(* Logix 5000 AddOnInstructionDefinition export AMCI_5034_PTO_AM_MAFR; software revision 37.00 *)

TYPE AMCI_5034_PTO_AM_Input_Data :
STRUCT
   ConnectionFaulted : DINT;
   MovingCW : BOOL;
   MovingCCW : BOOL;
   InHoldState : BOOL;
   Stopped : BOOL;
   AtHome : BOOL;
   Accelerating : BOOL;
   Decelerating : BOOL;
   MoveComplete : BOOL;
   HomeInvalid : BOOL;
   InvalidProfile : BOOL;
   PositionInvalid : BOOL;
   InputError : BOOL;
   CommandError : BOOL;
   ConfigurationError : BOOL;
   ModuleOK : BOOL;
   GeneralPurposeOutputStatus : BOOL;
   Input1Active : BOOL;
   Input2Active : BOOL;
   Input3Active : BOOL;
   Input4Active : BOOL;
   bit_20_reserved : BOOL;
   bit_21_reserved : BOOL;
   bit_22_reserved : BOOL;
   EncoderFollowerMode : BOOL;
   BlendMoveRunning : BOOL;
   BlendMoveAcknowledge : BOOL;
   MinimumRegistrationProgrammed : BOOL;
   EncoderMotionDirection : BOOL;
   MultipleInputsWithSameFunction : BOOL;
   FSCExceedsNumberOfDataBits : BOOL;
   AbsoluteEncoderSetupError : BOOL;
   bit_31_reserved : BOOL;
   CurrentPosition : DINT;
   EncoderPosition : DINT;
   CapturedPosition : DINT;
END_STRUCT
END_TYPE

TYPE AMCI_5034_PTO_AM_Output_Data :
STRUCT
   Command_Word : DINT;
   TargetPosition : DINT;
   TargetVelocity : UDINT;
   Acceleration : DINT;
   Deceleration : DINT;
END_STRUCT
END_TYPE

ADD_ON_INSTRUCTION AMCI_5034_PTO_AM_MAFR   (* revision 1.0, vendor AMCI, ExecuteEnableInFalse *)
// AMCI Reset Errors
// Revision note:
// 10/01/2025 Initial Release
// Help:
// MOTION AXIS FAULT RESET:   Resets Command and Input Errors.  It will also reset the Move Complete Status Bit.
// AXIS INPUT DATA:  Input data from the AMCI 5034-PTO-AM.   Uses the AMCI_5034_PTO_Input_Data User Defined Data Type.
// AXIS OUTPUT DATA; Output data from the AOI to the AMCI 5034-PTO-AM.    Uses the AMCI_5034_PTO_Output_Data User Defined Data Type.
// EN (Enable) Set when rung is true, Reset when rung is false
// DN (Done) Set when command is sent to the motion device.  Reset when the rung is false.
// ER (Error) Set when a command or input error failed to clear.  Reset when the rung is false.
VAR_IN_OUT
   Axis_Input_Data : AMCI_5034_PTO_AM_Input_Data; {required}
   Axis_Output_Data : AMCI_5034_PTO_AM_Output_Data; {required}
END_VAR
VAR_OUTPUT
   EN : BOOL; {visible}   // set when rung with AOI is true
   DN : BOOL; {access Read Only, visible}   // set when reset error command sent to motion axis
   ER : BOOL; {access Read Only, visible}   // set when reset error command did not clear the error
END_VAR
VAR
   command_data_block : DINT[5];
        [0]   // Command Bits MSW
        [1]   // Command Bits LSW
        [2]   // Upper Target Position
        [3]   // Lower Target Position
        [4]   // Upper Programmed Speed
END_VAR

ROUTINE EnableInFalse   (* ladder *)
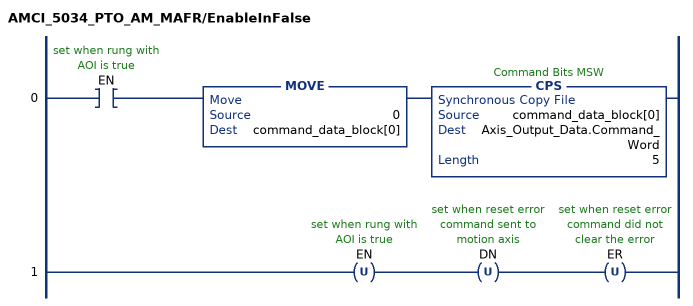
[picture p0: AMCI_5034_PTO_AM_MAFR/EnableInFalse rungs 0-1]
   0: XIC(EN)MOVE(0,command_data_block[0])CPS(command_data_block[0],Axis_Output_Data.Command_Word,5);
   1: OTU(EN)OTU(DN)OTU(ER);
END_ROUTINE

ROUTINE Logic   (* ladder *)
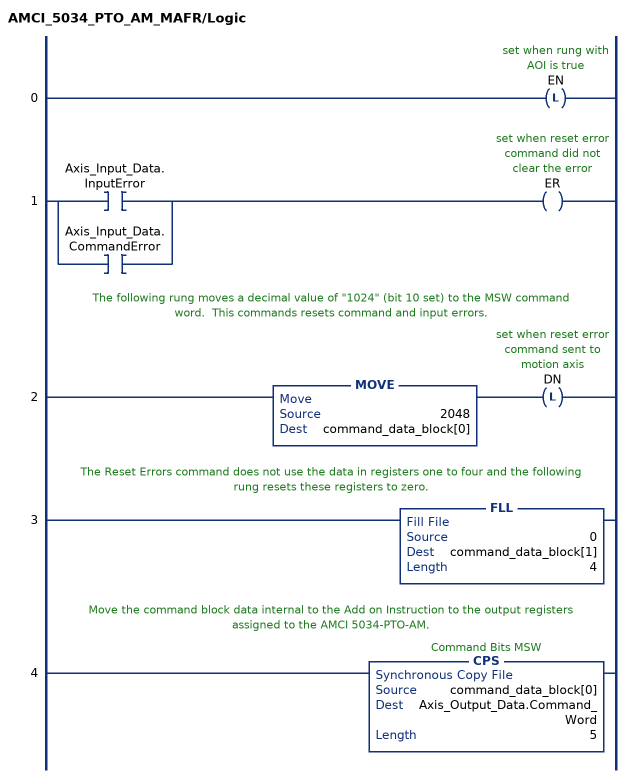
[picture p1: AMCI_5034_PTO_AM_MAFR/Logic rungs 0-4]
   0: OTL(EN);
   1: [XIC(Axis_Input_Data.InputError) ,XIC(Axis_Input_Data.CommandError) ]OTE(ER);
   // The following rung moves a decimal value of "1024" (bit 10 set) to the MSW command word.  This commands resets command and input errors.
   2: MOVE(2048,command_data_block[0])OTL(DN);
   // The Reset Errors command does not use the data in registers one to four and the following rung resets these registers to zero.
   3: FLL(0,command_data_block[1],4);
   // Move the command block data internal to the Add on Instruction to the output registers assigned to the AMCI 5034-PTO-AM.
   4: CPS(command_data_block[0],Axis_Output_Data.Command_Word,5);
END_ROUTINE
END_ADD_ON_INSTRUCTION
